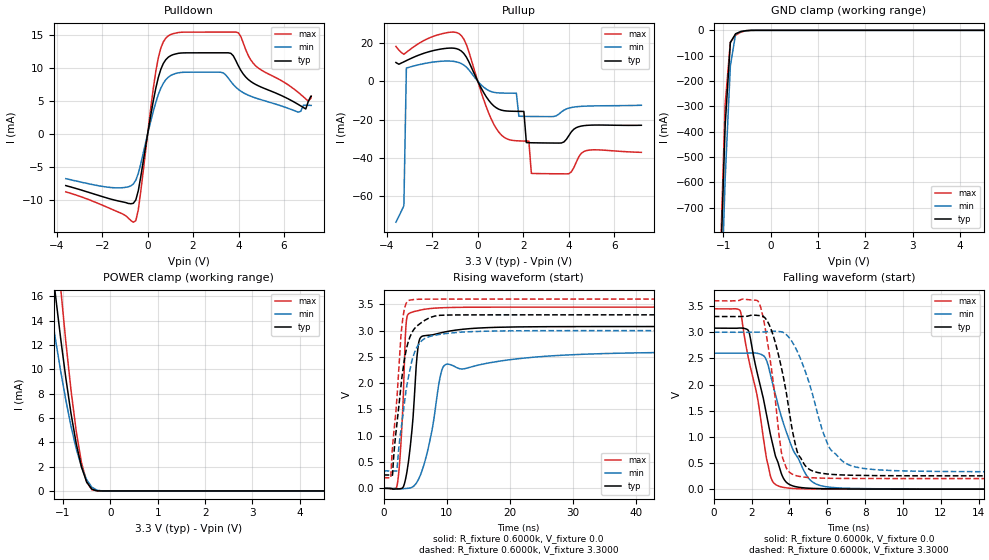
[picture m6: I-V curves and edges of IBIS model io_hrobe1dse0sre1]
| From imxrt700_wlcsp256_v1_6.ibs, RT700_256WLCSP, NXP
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[Model] io_hrobe1dse0sre1
|   Model io_hrobe1dse0sre1
| This model was characterised for following simulation conditions:
| External (pad) voltage:
|   - Typ: 3.3V,   - Min: 3.0V,   - Max: 3.6V
| Library cells for typ/min/max conditions are connected as defined below:
|  PAD_IO - External Pad
|  ipp_do - Core Input
|  ipp_obe - Output Buffer Enable
|  ASRCN3V3[3] - NC
|  ASRCN3V3[4] - NC
|  ASRCP3V3[4] - NC
|  REFAPBIAS3V3 - gnde
|  REFBAMPL3V3 - vdd1v8
|  REFCAMPH3V3 - vdd1v8
|  REFDNBIAS3V3 - vdd1v8
|  REFH3V3 - REFH3V3
|  REFL3V3 - REFL3V3
|  gnde - gnde
|  ipp_dse - gnde
|  ipp_ina235_3v - NC
|  ipp_ina40_3v - NC
|  ipp_ina_mux - NC
|  ipp_ind - NC
|  ipp_ind_1p8v - NC
|  ipp_ind_3v - NC
|  ipp_sre - vdd
|  vdd - vdd
|  vdd1v8 - vdd1v8
|  vdda - vdde3v3
|  vdde3v3 - vdde3v3
| All other pins connected to ground
Model_type I/O
Polarity   Non-Inverting
Enable   Active-High
Vinl =   0.9900V
Vinh =   2.3100V
Vmeas =  1.6500V
Cref =   15.0000pF
Rref =   0.6000k
Vref =   0.0V
C_comp   4.0008pF   3.8189pF   4.1206pF
|C_comp_pullup   0.5641pF   0.7338pF   0.4700pF
|C_comp_pulldown   2.1155pF   2.2137pF   1.8991pF
[Model Spec]
| variable   typ   min   max
Vinh   2.3100V   NA   NA
Vinl   0.9900V   NA   NA
Vref   0.0V   0.0V   0.0V
Cref   15.0000pF   15.0000pF   15.0000pF
Rref   0.6000k   0.6000k   0.6000k
[Receiver Thresholds]
Vcross_high  =   0.0V
Vcross_low  =   0.0V
Vdiff_ac  =   0.0V
Vdiff_dc  =   0.0V
Tdiffslew_ac  =   0.0S
[Temperature Range]   25.0000   0.1250k   -40.0000
[Voltage Range]   3.3000V   3.0000V   3.6000V
[Pullup Reference]   3.3000V   3.0000V   3.6000V
[Pulldown Reference]   0.0V   0.0V   0.0V
[POWER Clamp Reference]   3.3000V   3.0000V   3.6000V
[GND Clamp Reference]   0.0V   0.0V   0.0V
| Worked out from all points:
|   slope of the pulldown table from 0 to 0.495 V, typ, clamps not added: 56.2 ohm
|   slope of the pullup table from 0 to 0.495 V, typ, clamps not added: 48.6 ohm
|   GND clamp passes 1 mA (typ) near -0.49 V on its own axis
|   POWER clamp passes 1 mA (typ) near -0.52 V on its own axis
|   rising waveform, R_fixture 0.6000k, V_fixture 0.0: 20-80 % time 1.2ns typ, 2.33ns min, 732ps max; typ from 0 V to 3.08 V
|   rising waveform, R_fixture 0.6000k, V_fixture 3.3000: 20-80 % time 1.91ns typ, 2.09ns min, 1.29ns max; typ from 0.254 V to 3.3 V
|   falling waveform, R_fixture 0.6000k, V_fixture 0.0: 20-80 % time 1.13ns typ, 1.49ns min, 1.04ns max; typ from 3.08 V to 0 V
|   falling waveform, R_fixture 0.6000k, V_fixture 3.3000: 20-80 % time 973ps typ, 1.4ns min, 713ps max; typ from 3.3 V to 0.254 V
[Pulldown]
|Voltage   I(typ)   I(min)   I(max)
-3.6V     -7.76mA    -6.72mA    -8.7mA
-1.4V     -9.994mA   -8.101mA   -11.59mA
-520mV    -9.932mA   -6.949mA   -13.06mA
-410mV    -8.543mA   -5.943mA   -11.42mA
470mV     8.52mA     5.95mA     11.5mA
1.02V     11.84mA    8.845mA    15.02mA
3.22V     12.26mA    9.331mA    15.38mA
3.99V     10.32mA    6.757mA    15.29mA
4.76V     7.477mA    5.441mA    10.28mA
6.63V     4.475mA    3.308mA    6.287mA
6.96V     3.791mA    4.357mA    5.305mA
7.2V      5.701mA    4.331mA    5.72mA
[Pullup]
|Voltage   I(typ)   I(min)   I(max)
-3.6V     9.752mA    -73.55mA   18.1mA
-3.25V    10.1mA     -64.94mA   14.02mA
-3.14V    10.73mA    6.826mA    15.05mA
-720mV    15.71mA    9.188mA    23.77mA
820mV     -13.92mA   -6.016mA   -24.78mA
1.7V      -15.72mA   -6.277mA   -31.08mA
1.81V     -15.74mA   -18.26mA   -31.14mA
2.03V     -15.78mA   -18.35mA   -31.22mA
2.14V     -32.03mA   -18.37mA   -31.25mA
2.25V     -32.08mA   -18.39mA   -31.27mA
2.36V     -32.12mA   -18.41mA   -48.1mA
7.2V      -22.99mA   -12.56mA   -37.11mA
[GND_clamp]
|Voltage   I(typ)   I(min)   I(max)
-3.6V     -19.67A    -19.55A    -20.65A
-1.07V    -1.013A    -1.224A    -956.3mA
-960mV    -377.1mA   -587.4mA   -291.7mA
-850mV    -48.21mA   -140.8mA   -46.94mA
-740mV    -13.57mA   -15.59mA   -19.22mA
-630mV    -5.137mA   -4.351mA   -7.235mA
-520mV    -1.276mA   -1.53mA    -1.554mA
-300mV    -4.403uA   -32.47uA   -997nA
7.2V      0A         0A         0A
[POWER_clamp]
|Voltage   I(typ)   I(min)   I(max)
-3.6V     102.5mA    81.21mA    131.1mA
-1.38V    23.81mA    18.18mA    31.78mA
-1.27V    19.88mA    15.26mA    26.56mA
-1.16V    16.12mA    12.48mA    21.52mA
-1.05V    12.56mA    9.868mA    16.71mA
-830mV    6.344mA    5.304mA    8.253mA
-720mV    3.878mA    3.458mA    4.888mA
-610mV    1.973mA    1.979mA    2.327mA
-500mV    725uA      918.2uA    733.4uA
-390mV    144.3uA    301.5uA    95.95uA
-170mV    198.2nA    4.056uA    20.28nA
7.2V      0A         0A         0A
[Ramp]
| variable   typ   min   max
dV/dt_r  1.8464/1.2036n   1.5570/2.3301n   2.0681/0.7317n
dV/dt_f  1.8274/0.9727n   1.6009/1.4018n   2.0384/0.7125n
R_load = 0.6000k
[Rising Waveform]
R_fixture= 0.6000k
V_fixture= 0.0
V_fixture_min= 0.0
V_fixture_max= 0.0
|time   V(typ)   V(min)   V(max)
0s        180nV      2.945uV    139nV
2.212ns   -11.26mV   -14.85mV   109mV
2.86ns    -1.329mV   -9.127mV   1.105V
3.534ns   210mV      -4.265mV   3.082V
4.165ns   732.6mV    5.566mV    3.335V
5.673ns   2.825V     206.6mV    3.386V
7.502ns   2.915V     1.002V     3.421V
9.07ns    2.958V     2.18V      3.434V
9.877ns   2.979V     2.357V     3.437V
60ns      3.077V     2.595V     3.447V
[Rising Waveform]
R_fixture= 0.6000k
V_fixture= 3.3000
V_fixture_min= 3.0000
V_fixture_max= 3.6000
|time   V(typ)   V(min)   V(max)
0s        254.3mV    331.8mV    202.7mV
1.125ns   253.8mV    331.7mV    206mV
1.409ns   254.2mV    331.3mV    798.8mV
2.091ns   1.201V     330.8mV    1.683V
2.824ns   2.048V     1.181V     3.006V
3.298ns   2.453V     1.629V     3.415V
3.917ns   2.793V     2.105V     3.57V
5.741ns   3.131V     2.769V     3.597V
10.03ns   3.296V     2.948V     3.599V
60ns      3.3V       3V         3.6V
[Falling Waveform]
R_fixture= 0.6000k
V_fixture= 0.0
V_fixture_min= 0.0
V_fixture_max= 0.0
|time   V(typ)   V(min)   V(max)
0s        3.077V     2.599V     3.447V
1.385ns   3.079V     2.598V     3.415V
1.839ns   3.023V     2.597V     2.491V
2.306ns   2.208V     2.597V     1.76V
2.659ns   1.664V     2.541V     886.6mV
2.999ns   1.037V     2.182V     246.7mV
3.767ns   160.9mV    1.166V     28.92mV
5.024ns   18.09mV    203.5mV    4.316mV
6.424ns   5.602mV    27.69mV    904.4uV
60ns      675.2nV    2.182uV    424.3nV
[Falling Waveform]
R_fixture= 0.6000k
V_fixture= 3.3000
V_fixture_min= 3.0000
V_fixture_max= 3.6000
|time   V(typ)   V(min)   V(max)
0s        3.3V       3V         3.6V
2.379ns   3.318V     3.001V     3.571V
2.906ns   3.16V      3.013V     2.662V
3.613ns   2.259V     3.004V     633.5mV
4.296ns   882.8mV    2.72V      265mV
4.684ns   537.5mV    2.403V     234.4mV
6.153ns   284.8mV    769.4mV    207.4mV
7.032ns   268.6mV    484.3mV    204.5mV
8.173ns   260.4mV    384.3mV    203.2mV
60ns      254.3mV    331.8mV    202.7mV
